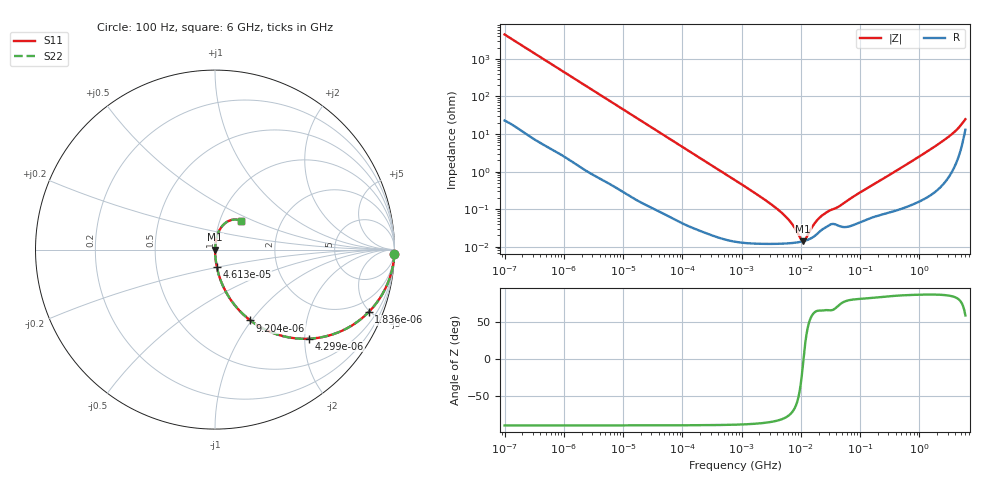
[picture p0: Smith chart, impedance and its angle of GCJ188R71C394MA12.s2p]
!Murata Part Number: GCJ188R71C394MA12
!These Parameters are Measured in Series Mode Connection
!Data Generated on Mar 13, 2026
!  o--ll--o
!Port1  Port2
!  o------o
!Operation Temp=25[degC], DC Bias Voltage=0[V]
!Freq. Start=100[Hz] Stop=6[GHz] 401[Steps]
# Hz S RI R 50
!Freq.(Hz) S11(Real) S11(Imag) S21(Real) S21(Imag) S12(Real) S12(Imag) S22(Real) S22(Imag)
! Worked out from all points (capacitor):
!   401 points, 100 Hz to 6 GHz, reference 50 ohm
!   read as one part in series: C = 356 nF near 109 Hz
!   lowest |Z| = 14.1 mohm at 10.87 MHz (marker M1)
!   series resonance near 11.12 MHz, so ESL is about 580 pH
!   S11 on the Smith chart (normalised r, x): 100 Hz: 1, -89; 1.836 kHz: 1.03, -4.91; 4.299 kHz: 1.01, -2.10; 9.204 kHz: 1.01, -0.99; 46.13 kHz: 1.00, -0.20; 6 GHz: 1.26, +0.42
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100  0.9994 -0.0224  0.000617 0.0224  0.000617 0.0224  0.9994 -0.0224
524  0.9859 -0.1151  0.0141 0.1151  0.0141 0.1151  0.9859 -0.1151
1836  0.8563 -0.3481  0.1437 0.3481  0.1437 0.3481  0.8563 -0.3481
2008  0.8331 -0.3702  0.1669 0.3702  0.1669 0.3702  0.8331 -0.3702
4299  0.5248 -0.4964  0.4752 0.4964  0.4752 0.4964  0.5248 -0.4964
9204  0.1968 -0.3944  0.8032 0.3944  0.8032 0.3944  0.1968 -0.3944
17227  0.0664 -0.2458  0.9336 0.2458  0.9336 0.2458  0.0664 -0.2458
40335  0.0135 -0.1114  0.9865 0.1114  0.9865 0.1114  0.0135 -0.1114
46134  0.0104 -0.0978  0.9896 0.0978  0.9896 0.0978  0.0104 -0.0978
774597  0.000171 -0.00593  0.9998 0.00593  0.9998 0.00593  0.000171 -0.00593
4643984  0.000121 -0.000823  0.9999 0.000823  0.9999 0.000823  0.000121 -0.000823
6644369  0.000125 -0.000449  0.9999 0.000449  0.9999 0.000449  0.000125 -0.000449
9941735  0.000136 -9.38e-05  0.9999 9.38e-05  0.9999 9.38e-05  0.000136 -9.38e-05
1.087309e7  0.00014 -1.86e-05  0.9999 1.86e-05  0.9999 1.86e-05  0.00014 -1.86e-05
1.243624e7  0.000149 9.44e-05  0.9999 -9.44e-05  0.9999 -9.44e-05  0.000149 9.44e-05
1.555665e7  0.000175 0.000289  0.9998 -0.000289  0.9998 -0.000289  0.000175 0.000289
1.946e7  0.00023 0.000489  0.9998 -0.000489  0.9998 -0.000489  0.00023 0.000489
2.662322e7  0.000333 0.000734  0.9997 -0.000734  0.9997 -0.000734  0.000333 0.000734
3.124326e8  0.00088 0.00808  0.9991 -0.00808  0.9991 -0.00808  0.00088 0.00808
2.34314e9  0.00764 0.06  0.9924 -0.06  0.9924 -0.06  0.00764 0.06
4.385646e9  0.0362 0.1263  0.9638 -0.1263  0.9638 -0.1263  0.0362 0.1263
6e9  0.145 0.16  0.855 -0.16  0.855 -0.16  0.145 0.16
